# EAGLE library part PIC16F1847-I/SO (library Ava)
IC, 18 Pin Flash Microcontrollers with XLP Technology-SOIC-18
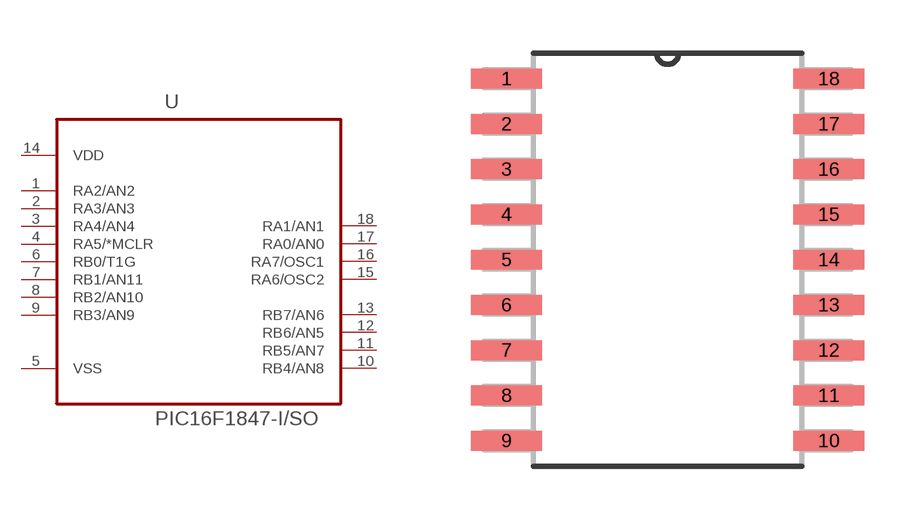
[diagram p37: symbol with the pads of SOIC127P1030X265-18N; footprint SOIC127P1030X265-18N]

Designator prefix U

## PIC16F1847-I/SO (MPN: PIC16F1847-I/SO; OC_FARNELL: 1971870; OC_NEWARK: 23T3107; PACKAGE: SOIC-18; SUPPLIER: Microchip)  [SOIC127P1030X265-18N]
1  RA2/AN2
2  RA3/AN3
3  RA4/AN4
4  RA5/*MCLR
5  VSS  pwr
6  RB0/T1G
7  RB1/AN11
8  RB2/AN10
9  RB3/AN9
10  RB4/AN8
11  RB5/AN7
12  RB6/AN5
13  RB7/AN6
14  VDD  pwr
15  RA6/OSC2
16  RA7/OSC1
17  RA0/AN0
18  RA1/AN1

## Footprint SOIC127P1030X265-18N (pad centres in mm)
smd 1.981 x 0.559: 1 -4.521,5.08; 2 -4.521,3.81; 3 -4.521,2.54; 4 -4.521,1.27; 5 -4.521,0; 6 -4.521,-1.27; 7 -4.521,-2.54; 8 -4.521,-3.81; 9 -4.521,-5.08; 10 4.521,-5.08; 11 4.521,-3.81; 12 4.521,-2.54; 13 4.521,-1.27; 14 4.521,0; 15 4.521,1.27; 16 4.521,2.54; 17 4.521,3.81; 18 4.521,5.08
